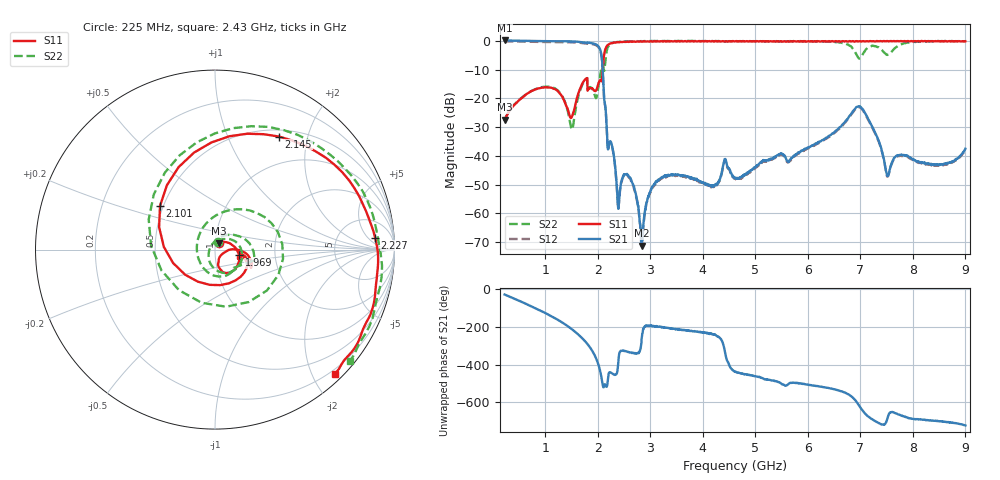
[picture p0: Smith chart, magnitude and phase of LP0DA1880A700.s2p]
!Agilent Technologies,E8358A,US41080443,A.07.50.56
!Agilent E8358A: A.07.50.56
!Date: Tuesday, June 21, 2016 11:37:26
!Correction: S11(Full 2 Port(1,2))
!S21(Full 2 Port(1,2))
!S12(Full 2 Port(1,2))
!S22(Full 2 Port(1,2))
!S2P File: Measurements: S11, S21, S12, S22:
# Hz S  dB  R 50
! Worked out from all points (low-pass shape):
!   1601 points, 225 MHz to 9 GHz, reference 50 ohm
!   highest |S21| = 0.17 dB at 230.5 MHz (marker M1); lowest = -71.2 dB at 2.836 GHz (marker M2)
!   |S21| within 3 dB of the highest: start of sweep to 2.041 GHz
!   lowest |S11| = -27.4 dB at 225 MHz (marker M3), VSWR 1.09, Z = 52.2 + j3.75 ohm
!   |S11| at or under -10 dB: start of sweep to 2.093 GHz
!   |S22| runs from -30.9 to 0.0 dB; largest |S21 - S12| = 0.036
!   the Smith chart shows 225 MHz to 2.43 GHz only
!   S11 on the Smith chart (normalised r, x): 225 MHz: 1.04, +0.07; 1.969 GHz: 1.31, -0.08; 2.101 GHz: 0.48, +0.28; 2.145 GHz: 0.59, +1.55; 2.227 GHz: 12, +8; 2.43 GHz: 0.13, -2.35
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2.25e8  -27.44 57.6  0.16 -27.0  -0.14 -26.7  -27.38 69.6
2.304844e8  -27.28 56.6  0.17 -27.6  -0.14 -27.4  -27.16 68.8
9.160312e8  -16.34 -32.8  -0.05 -113.3  -0.35 -113.2  -16.14 -14.3
1.36575e9  -21.04 -78.4  -0.10 176.7  -0.40 176.8  -20.80 -101.9
1.508344e9  -26.38 -28.1  -0.15 148.4  -0.45 148.5  -30.88 152.6
1.689328e9  -15.46 -6.0  -0.42 104.6  -0.72 104.7  -15.87 25.8
1.969031e9  -17.17 -13.3  -1.24 -7.2  -1.55 -7.1  -19.89 178.9
2.100656e9  -8.16 141.6  -12.63 -156.2  -12.90 -156.1  -8.67 -38.2
2.144531e9  -2.81 60.5  -22.98 -148.2  -23.24 -148.1  -6.76 137.9
2.226797e9  -0.97 4.3  -35.03 -79.4  -35.34 -79.2  -1.26 28.4
2.429719e9  -0.34 -46.0  -50.88 31.4  -51.10 30.7  -0.21 -39.5
2.835562e9  -0.23 -85.9  -71.23 103.1  -71.00 85.0  -0.11 -87.9
3.153656e9  -0.13 -102.9  -48.36 161.5  -48.65 162.0  -0.02 -109.6
4.6125e9  -0.17 -143.3  -47.61 -74.9  -47.77 -76.9  -0.08 170.6
6.076828e9  -0.08 179.8  -36.36 -148.8  -36.82 -149.3  -0.21 71.5
6.740438e9  -0.14 165.2  -27.38 167.0  -27.70 167.5  -1.13 5.1
6.987234e9  -0.07 162.1  -22.72 98.4  -23.06 98.5  -6.12 -148.4
7.184672e9  -0.04 159.1  -28.35 37.8  -28.72 37.6  -2.02 76.1
7.382109e9  -0.03 156.9  -36.42 5.2  -36.79 5.5  -2.76 2.7
7.541156e9  -0.16 155.0  -46.26 57.1  -46.28 54.8  -4.69 -115.7
7.925062e9  -0.13 151.6  -40.32 36.3  -40.69 36.7  -0.55 106.9
9e9  -0.13 141.9  -37.50 -2.4  -37.80 -2.7  -0.10 50.3
